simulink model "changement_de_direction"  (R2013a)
settings: Solver=ode45  StartTime=0.0  StopTime=inf  RelTol=1e-3
libraries: simulink x1

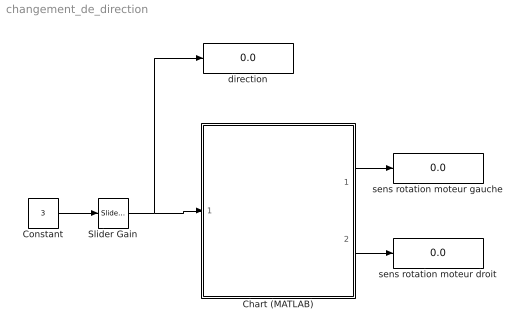
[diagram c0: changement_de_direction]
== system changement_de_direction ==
  Chart (MATLAB) : Stateflow chart  TreatAsAtomicUnit=on
  Constant : Constant  Value=3
  Slider Gain : simulink/Math Operations/Slider Gain  low=0  gain=0.5  high=1
  direction : Display
  sens rotation moteur droit : Display
  sens rotation moteur gauche : Display
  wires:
  Slider Gain/1 -> direction/1, Chart (MATLAB)/1(direction)
  Constant/1 -> Slider Gain/1
  Chart (MATLAB)/1(mg) -> sens rotation moteur gauche/1
  Chart (MATLAB)/2(md) -> sens rotation moteur droit/1
